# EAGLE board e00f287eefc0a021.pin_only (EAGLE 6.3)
REV: B

Size 24.13 x 15.24 mm. Coordinates in mm from the lower left corner, seen from the top.
Outline: 0,2.54 0,12.7 arc-90 2.54,15.24 21.59,15.24 arc-90 24.13,12.7 24.13,2.54 arc-90 21.59,0 2.54,0 arc-90 0,2.54
Copper layers (1*16): Top 0.035mm / dielectric 1.5mm / Bottom 0.035mm
Design rules "adafruit": minimum track width 8mil, minimum drill 15.5mil, track to track 8mil, track to pad 8mil, pad to pad 8mil, via to via 8mil, smd to smd 8mil, copper to edge 10mil, drill to drill 8mil, minimum pad ring 10mil, minimum via ring 8mil, stop-mask expansion 2mil, vias tented up to drill 20mil, thermal gap 10mil

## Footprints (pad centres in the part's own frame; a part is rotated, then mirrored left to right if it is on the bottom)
0805-NO = smd 1.3 x 1.5: 1 -0.95,0; 2 0.95,0
_0805 = smd 1.2 x 1.3: 1 -1.016,0; 2 1.016,0
FIDUCIAL_1MM = smd 1 x 1: 1 0,0
1X05_ROUND_70 = drill 1 pad 1.778 square: 1 -5.08,0 | drill 1 pad 1.778: 2 -2.54,0; 3 0,0; 4 2.54,0; 5 5.08,0
MSOP8_0.65MM = smd 0.4 x 1.4: 1 -0.975,-2.2; 2 -0.325,-2.2; 3 0.325,-2.2; 4 0.975,-2.2; 5 0.975,2.2; 6 0.325,2.2; 7 -0.325,2.2; 8 -0.975,2.2
MOUNTINGHOLE_2.0_PLATED = drill 2.2 pad 3: P$1 0,0
TRIMPOT_BOURNS_3303W = smd 1.2 x 1.2: 1 -1,-1.6; 3 1,-1.6 | smd 1.6 x 1.5: 2 0,1.65
TERMBLOCK_1X2-3.5MM = drill 1 pad 2.184: 1 1.8,0; 2 -1.7,0

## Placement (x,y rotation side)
C1  1uF  [0805-NO]  11.94,12.7 180 top
C2  1uF  [0805-NO]  6.86,9.65 180 top
C3  10uF  [0805-NO]  8.13,3.81 90 top
C4  220pF  [0805-NO]  14.48,2.54 180 top
C5  220pF  [0805-NO]  14.61,8.51 180 top
FB1  Ferrite  [_0805]  14.61,6.48 0 top
FB2  Ferrite  [_0805]  14.61,4.32 0 top
FID1  FIDUCIAL""  [FIDUCIAL_1MM]  18.29,7.24 0 top
FID2  FIDUCIAL""  [FIDUCIAL_1MM]  1.14,5.59 0 top
JP1  [1X05_ROUND_70]  3.05,7.62 90 top
R1  100  [0805-NO]  11.18,10.03 270 top
R2  100  [0805-NO]  7.75,7.62 0 top
R3  10K  [0805-NO]  6.35,4.57 90 top
U1  PAM8302AASCR  [MSOP8_0.65MM]  10.79,5.08 180 top
U$3  [SYMBOL_PLUS]  18.8,12.19 180 top
U$4  [SYMBOL_MINUS]  18.67,2.92 0 top
U$5  [ADAFRUIT_3.5MM]  17.02,9.4 90 top
U$6  [PCBFEAT-REV-040]  17.65,13.97 0 bottom
U$10  MOUNTINGHOLE2.0  [MOUNTINGHOLE_2.0_PLATED]  21.59,12.95 0 top
U$11  MOUNTINGHOLE2.0  [MOUNTINGHOLE_2.0_PLATED]  21.59,2.29 0 top
VR1  10K trim  [TRIMPOT_BOURNS_3303W]  7.62,12.7 270 top
X1  [TERMBLOCK_1X2-3.5MM]  20.45,7.49 90 top

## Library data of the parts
C1-C5 FB1 FB2 JP1 R2 U1 U$3-U$6 VR1 X1 = microbuilder
FID1 FID2 U$10 U$11 = microbuilder; BOM: EXCLUDE
R1 R3 = microbuilder; COMPANY: ADAFRUIT INDUSTRIES; DRAWN: KTOWN; REV: A

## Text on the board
tPlace: PAM8302A | A+ | A- | Vol | SD | 4-8Ω | Vin | Gnd | 2.5W ClassD Amp
bPlace: Audio In+ | (diff in) | Audio In- | Max 24dB Gain | Shutdown | Mono Class D Amp | adafruit! | 4-8Ω Load | 2-5VDC | Ground | PAM8302A

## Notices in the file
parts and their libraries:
microbuilder: This work is placed in the public domain, and may be freely used for commercial and non-commercial work with the following conditions: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
